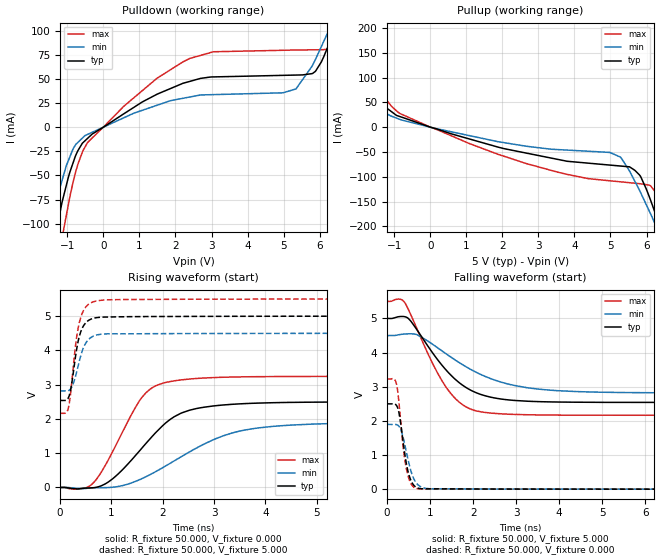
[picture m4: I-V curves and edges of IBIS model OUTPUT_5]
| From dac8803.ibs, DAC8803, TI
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|   Output OUTPUT 5 Model
[Model]   OUTPUT_5
Model_type Output
|Signal SDO(20) pin
Polarity   Non-Inverting
Enable   Active-Low
Vmeas = 2.5
Vref = 2.5
Cref = 15pF
Rref = 50
|   typ   min   max
|   (nom PVT)   (Fast PVT)   (slow PVT)
|Average
C_comp   3.468e-12   3.241e-12   3.773e-12
|ON state : BUFFER OUTPUT TURNED HIGH
|C_comp   3.137e-12   3.078e-12   3.467e-12
|OFF state: BUFFER in HIGH IMPEDANCE for IOs and 3-state,
|This is BUFFER in LOW state for OUTPUT only type
|C_comp   3.470e-12   3.404e-12   4.408e-12
| Where   nom PVT is  Nominal Process, 5.0V, 25C
|   Fast PVT is Strong Process, 5.5V, -40C
|   Slow PVT is Weak Process, 4.5V, 85C
[Voltage Range]   5   4.5   5.5
|Ambient Temperature   25   85   -40
|Junction Temperature
[Temperature Range]   25   85   -40
[Pullup Reference]   5   4.5   5.5
[Pulldown Reference]   0   0   0
[Power Clamp Reference]   5   4.5   5.5
[GND Clamp Reference]   0   0   0
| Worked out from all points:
|   slope of the pulldown table from 0 to 0.75 V, typ, clamps not added: 41.2 ohm
|   slope of the pullup table from 0 to 0.75 V, typ, clamps not added: 44.2 ohm
|   falling waveform, R_fixture 50.000, V_fixture 5.000: 20-80 % time 991ps typ, 1.45ns min, 815ps max; typ from 5 V to 2.54 V
|   rising waveform, R_fixture 50.000, V_fixture 0.000: 20-80 % time 954ps typ, 1.45ns min, 695ps max; typ from 0 V to 2.5 V
|   rising waveform, R_fixture 50.000, V_fixture 5.000: 20-80 % time 168ps typ, 198ps min, 167ps max; typ from 2.54 V to 5 V
|   falling waveform, R_fixture 50.000, V_fixture 0.000: 20-80 % time 183ps typ, 223ps min, 169ps max; typ from 2.5 V to 0 V
[Pulldown]
|   Voltage   I(typ)   I(min)   I(max)
-5V       -968.6mA   -712.6mA   -1.388A
-1.491V   -146.2mA   -103.8mA   -211mA
-1.288V   -104.6mA   -73.72mA   -149.4mA
-1.15V    -78.13mA   -55.53mA   -115.2mA
-780mV    -30.33mA   -18.66mA   -47.94mA
-440.5mV  -11.66mA   -7.558mA   -16.02mA
2.397V    47.37mA    31.21mA    71.15mA
5.341V    53.92mA    39.54mA    79.87mA
5.875V    57.55mA    69.52mA    80.06mA
6.346V    94.9mA     107.8mA    81.39mA
6.676V    127.8mA    134.7mA    109.7mA
10V       427.8mA    374.8mA    505.9mA
[Pullup]
|   Voltage   I(typ)   I(min)   I(max)
-5V       346.7mA    291.1mA    424.8mA
-3.495V   240.7mA    197.6mA    301.5mA
-2.684V   171.5mA    138.7mA    218mA
-1.545V   64.06mA    49.25mA    85.22mA
-842mV    21.3mA     15.55mA    27.52mA
2.656V    -52.23mA   -38.42mA   -73.28mA
5.278V    -78.44mA   -60.45mA   -110.3mA
5.825V    -98.36mA   -130.5mA   -114.2mA
6.11V     -147mA     -174.6mA   -118.1mA
6.374V    -201.9mA   -217.9mA   -151.3mA
6.66V     -264.4mA   -266.1mA   -221.6mA
10V       -1.058A    -861.1mA   -1.342A
[Ramp]
R_load = 50
|   typ   min   max
dV/dt_r   1.52778/9.54322e-10   1.14141/1.44559e-09   1.94609/6.94937e-10
dV/dt_f   1.47618/9.90074e-10   1.00885/1.45077e-09   2.00144/8.15227e-10
[Falling Waveform]
R_fixture = 50.000
V_fixture = 5.000
V_fixture_min = 4.500
V_fixture_max = 5.500
C_fixture = 0.000
|  time   V(typ)   V(min)   V(max)
0s        5V         4.5V       5.5V
400ps     5.054V     4.544V     5.485V
700ps     4.66V      4.522V     4.684V
1.05ns    4.009V     4.251V     3.707V
1.35ns    3.522V     3.986V     3.03V
1.675ns   3.122V     3.709V     2.552V
2.025ns   2.851V     3.454V     2.31V
2.825ns   2.614V     3.076V     2.196V
3.8ns     2.556V     2.899V     2.171V
8.975ns   2.54V      2.819V     2.164V
[Rising Waveform]
R_fixture = 50.000
V_fixture = 0.000
V_fixture_min = 0.000
V_fixture_max = 0.000
C_fixture = 0.000
|  time   V(typ)   V(min)   V(max)
0s        0V         1.864nV    1.45nV
450ps     -24.38mV   -33.66mV   -26.54mV
650ps     -7.498mV   -12.34mV   138mV
1.025ns   254.8mV    6.242mV    1.052V
1.55ns    1.072V     227.6mV    2.541V
1.775ns   1.457V     391.4mV    2.89V
2.05ns    1.873V     621.3mV    3.063V
2.65ns    2.301V     1.144V     3.18V
3.875ns   2.463V     1.74V      3.234V
8.975ns   2.499V     1.902V     3.243V
[Rising Waveform]
R_fixture = 50.000
V_fixture = 5.000
V_fixture_min = 4.500
V_fixture_max = 5.500
C_fixture = 0.000
|  time   V(typ)   V(min)   V(max)
0s        2.539V     2.818V     2.164V
125ps     2.549V     2.818V     2.187V
175ps     2.668V     2.836V     2.422V
225ps     3.026V     2.925V     3.041V
300ps     3.825V     3.245V     4.15V
350ps     4.264V     3.54V      4.646V
400ps     4.538V     3.834V     4.956V
500ps     4.81V      4.217V     5.27V
675ps     4.948V     4.433V     5.433V
8.975ns   5V         4.5V       5.5V
[Falling Waveform]
R_fixture = 50.000
V_fixture = 0.000
V_fixture_min = 0.000
V_fixture_max = 0.000
C_fixture = 0.000
|  time   V(typ)   V(min)   V(max)
0s        2.499V     1.896V     3.226V
150ps     2.502V     1.896V     3.236V
225ps     2.444V     1.889V     3.058V
300ps     2.078V     1.802V     2.231V
375ps     1.379V     1.512V     1.234V
450ps     745.9mV    1.086V     600mV
550ps     271.5mV    558.4mV    174.9mV
700ps     38.68mV    151.9mV    15.6mV
1.125ns   9.509mV    8.47mV     12.13mV
8.975ns   0V         486.6uV    106.2uV
